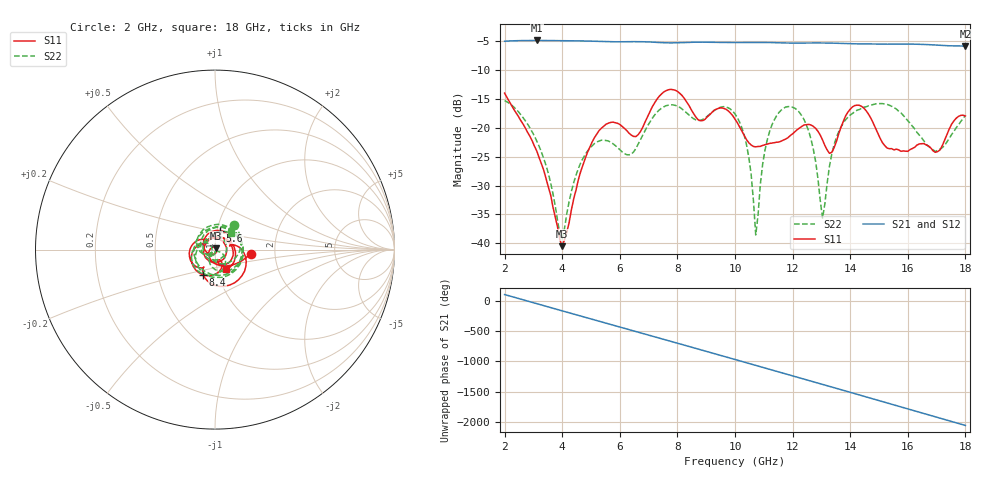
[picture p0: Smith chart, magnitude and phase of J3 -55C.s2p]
!Agilent Technologies,E8363B,SG43030131,A.07.50.48
!Agilent E8363B: A.07.50.48
!Date: Wednesday, December 17, 2025 22:25:37
!Correction: S11(Full 2 Port(1,2))
!S21(Full 2 Port(1,2))
!S12(Full 2 Port(1,2))
!S22(Full 2 Port(1,2))
!S2P File: Measurements: S11, S21, S12, S22:
# Hz S  dB  R 50
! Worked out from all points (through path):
!   201 points, 2 GHz to 18 GHz, reference 50 ohm
!   highest |S21| = -4.89 dB at 3.12 GHz (marker M1); lowest = -5.9 dB at 18 GHz (marker M2)
!   group delay of S21, straight-line fit = 373 ps
!   lowest |S11| = -40.5 dB at 4 GHz (marker M3), VSWR 1.02, Z = 50.7 + j0.667 ohm
!   |S11| at or under -10 dB: start of sweep to end of sweep
!   |S22| runs from -39.2 to -15.3 dB; largest |S21 - S12| = 0.0021
!   S11 on the Smith chart (normalised r, x): 2 GHz: 1.49, -0.07; 5.6 GHz: 1.03, +0.22; 8.4 GHz: 0.84, -0.25; 18 GHz: 1.10, -0.25
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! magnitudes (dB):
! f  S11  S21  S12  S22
! 2 GHz  -14.0  -5.0  -5.0  -15.3
! 3.12 GHz  -24.0  -4.9  -4.9  -22.3
! 4 GHz  -40.5  -4.9  -4.9  -39.2
! 4.72 GHz  -26.4  -5.0  -5.0  -25.3
! 5.6 GHz  -19.2  -5.1  -5.1  -22.3
! 6.56 GHz  -21.5  -5.1  -5.1  -23.6
! 7.36 GHz  -14.6  -5.2  -5.3  -17.0
! 8.4 GHz  -16.1  -5.2  -5.2  -17.8
! 10 GHz  -18.5  -5.3  -5.3  -17.6
! 10.48 GHz  -22.6  -5.2  -5.2  -25.1
! 10.72 GHz  -23.3  -5.2  -5.2  -38.5
! 11.04 GHz  -22.9  -5.2  -5.2  -23.9
! 11.44 GHz  -22.5  -5.3  -5.3  -18.0
! 12.16 GHz  -20.3  -5.4  -5.4  -16.9
! 12.72 GHz  -19.8  -5.3  -5.3  -23.7
! 13.04 GHz  -22.1  -5.3  -5.3  -35.6
! 13.36 GHz  -24.2  -5.4  -5.4  -24.6
! 13.76 GHz  -18.9  -5.4  -5.4  -19.1
! 14.4 GHz  -16.3  -5.5  -5.5  -16.6
! 15.36 GHz  -23.6  -5.5  -5.5  -16.1
! 16.96 GHz  -24.2  -5.7  -5.7  -24.1
! 18 GHz  -18.0  -5.9  -5.9  -17.9
